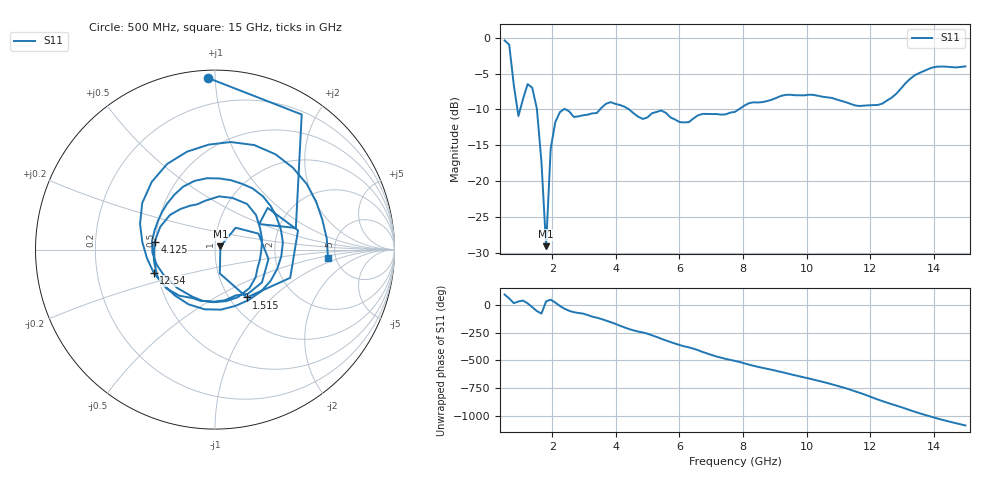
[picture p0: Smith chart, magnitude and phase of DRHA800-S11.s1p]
# Hz S DB R 50
! HP 8720B Vector Network Analyzer
! S-Parameter: S11
! Start Frequency: 500 MHz
! Stop Frequency: 15000 MHz
! Number of Points: 101
! Date: 26-Mar-2022 10:33:36
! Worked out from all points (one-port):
!   101 points, 500 MHz to 15 GHz, reference 50 ohm
!   lowest |S11| = -29.1 dB at 1.805 GHz (marker M1), VSWR 1.07, Z = 53.1 + j1.9 ohm
!   |S11| at or under -10 dB: 1.517 GHz to 2.359 GHz (842.3 MHz wide, 43.5 % of centre); 2.419 GHz to 3.502 GHz (1.083 GHz wide, 36.6 % of centre); 4.417 GHz to 7.867 GHz (3.45 GHz wide, 56.2 % of centre)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
!   S11 on the Smith chart (normalised r, x): 500 MHz: 0.04, +0.96; 1.515 GHz: 1.20, -0.71; 4.125 GHz: 0.49, +0.05; 12.54 GHz: 0.48, -0.14; 15 GHz: 4.31, -0.68
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5e8  -0.37 92.4
6.45e8  -0.97 57.3
7.9e8  -6.63 15.0
9.35e8  -10.92 30.0
1.08e9  -8.54 38.4
1.225e9  -6.47 13.0
1.37e9  -6.98 -20.6
1.515e9  -9.89 -56.3
1.66e9  -17.37 -78.6
1.805e9  -29.10 30.6
1.95e9  -15.50 46.6
2.385e9  -9.92 -35.0
3.545e9  -9.79 -127.5
4.125e9  -9.38 172.8
5.14e9  -10.53 85.6
6.01e9  -11.78 -1.3
6.88e9  -10.63 -77.6
7.75e9  -10.34 -144.2
8.62e9  -8.97 153.3
9.635e9  -8.02 86.6
1.065e10  -8.32 17.3
1.1375e10  -9.21 -42.6
1.1955e10  -9.43 -99.9
1.2535e10  -8.75 -159.3
1.326e10  -5.74 133.0
1.3985e10  -4.12 69.4
1.442e10  -4.04 35.6
1.5e10  -3.99 -4.3
